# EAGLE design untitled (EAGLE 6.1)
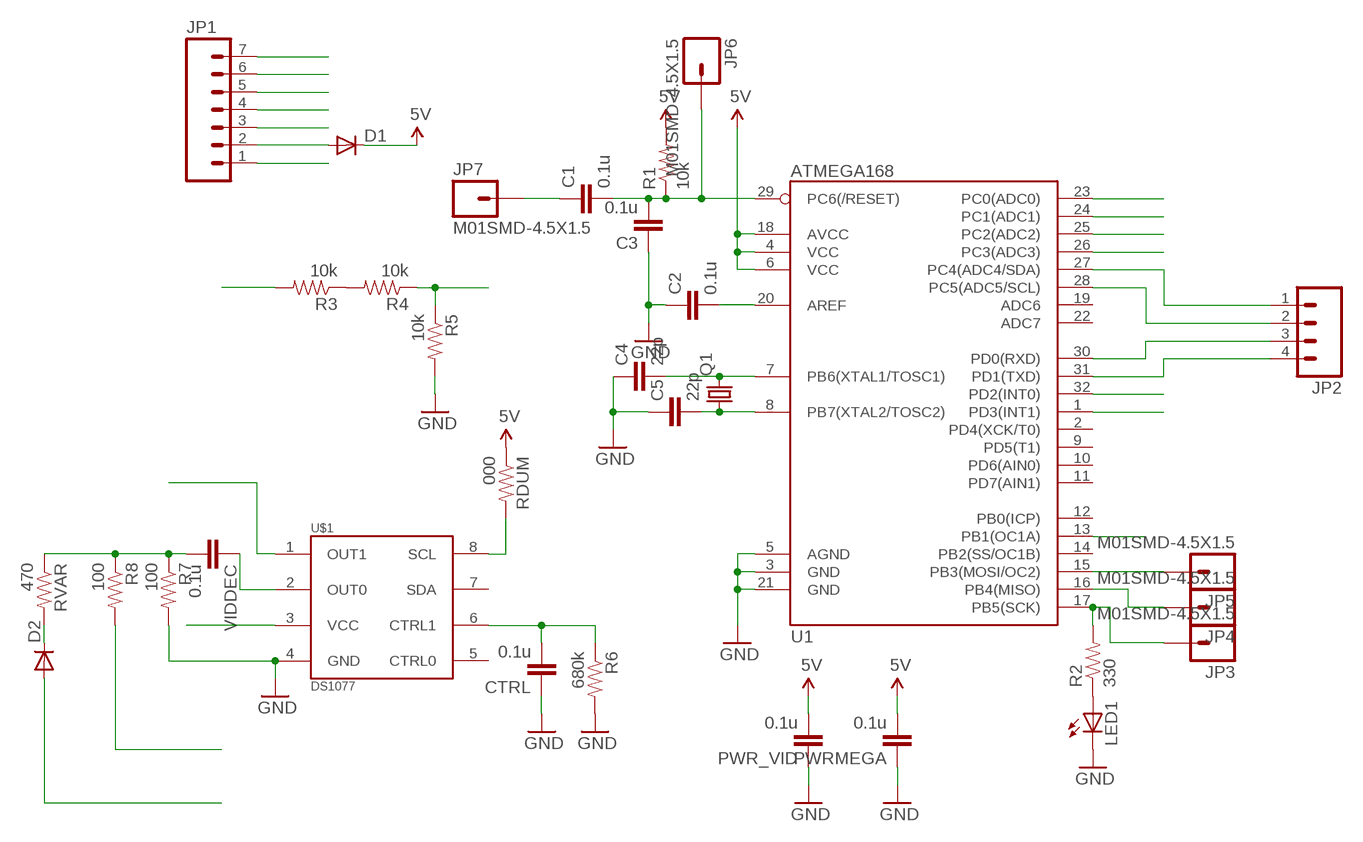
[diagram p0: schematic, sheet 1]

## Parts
C1  0.1u  CAP0805  [0805]
C2  0.1u  CAP0805  [0805]
C3  0.1u  CAP0805  [0805]
C4  22p  CAP0805  [0805]
C5  22p  CAP0805  [0805]
CTRL  0.1u  CAP0805  [0805]
D1  DIODESMA  [SMA-DIODE]
D2  DIODESMA  [SMA-DIODE]
JP1  M07  [1X07]
JP2  M04PTH  [1X04]
JP3  M01SMD-4.5X1.5  [PAD-1.5X4.5]
JP4  M01SMD-4.5X1.5  [PAD-1.5X4.5]
JP5  M01SMD-4.5X1.5  [PAD-1.5X4.5]
JP6  M01SMD-4.5X1.5  [PAD-1.5X4.5]
JP7  M01SMD-4.5X1.5  [PAD-1.5X4.5]
LED1  LED1206  [LED-1206]
PWR_VID  0.1u  CAP0805  [0805]
PWRMEGA  0.1u  CAP0805  [0805]
Q1  CRYSTAL10.5X4.8  [CRYSTAL-SMD-10.5X4.8-2PIN]
R1  10k  RESISTOR1206  [1206]
R2  330  RESISTOR1206  [1206]
R3  10k  RESISTOR1206  [1206]
R4  10k  RESISTOR1206  [1206]
R5  10k  RESISTOR1206  [1206]
R6  680k  RESISTOR1206  [1206]
R7  100  RESISTOR1206  [1206]
R8  100  RESISTOR1206  [1206]
RDUM  000  RESISTOR1206  [1206]
RVAR  470  RESISTOR1206  [1206]
U1  ATMEGA168  [TQFP32-08]
U$1  DS1077  [SO08]
VIDDEC  0.1u  CAP0805  [0805]

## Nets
5V: D1.C PWR_VID.2 PWRMEGA.2 R1.2 RDUM.1 U1.4(VCC) U1.6(VCC) U1.18(AVCC)
ADC0: JP1.4 U1.23(PC0(ADC0))
ADC2: JP1.5 U1.25(PC2(ADC2))
ADC3: JP1.6 U1.26(PC3(ADC3))
GND: C2.1 C3.1 C4.1 C5.1 CTRL.1 JP1.3 LED1.C PWR_VID.1 PWRMEGA.1 R5.2 R6.2 R7.2 U1.3(GND) U1.5(AGND) U1.21(GND) U$1.4(GND)
M1: U1.1(PD3(INT1)) U$1.3(VCC)
M13: R8.2 U1.13(PB1(OC1A))
M15: D2.A JP5.P$1 U1.15(PB3(MOSI/OC2))
M32: U1.32(PD2(INT0)) U$1.1(OUT1)
N$1: C2.2 U1.20(AREF)
N$2: C1.2 C3.2 JP6.P$1 R1.1 U1.29(PC6(/RESET))
N$3: C4.2 Q1.P$2 U1.7(PB6(XTAL1/TOSC1))
N$4: C5.2 Q1.P$1 U1.8(PB7(XTAL2/TOSC2))
N$5: JP2.1 U1.27(PC4(ADC4/SDA))
N$6: JP2.2 U1.28(PC5(ADC5/SCL))
N$7: JP2.3 U1.30(PD0(RXD))
N$8: JP2.4 U1.31(PD1(TXD))
N$9: LED1.A R2.1
N$10: JP3.P$1 R2.2 U1.17(PB5(SCK))
N$11: R3.1 R4.2
N$12: D1.A JP1.2
N$13: U$1.2(OUT0) VIDDEC.1
N$14: C1.1 JP7.P$1
N$15: RDUM.2 U$1.8(SCL)
N$16: JP4.P$1 U1.16(PB4(MISO))
N$19: CTRL.2 R6.1 U$1.6(CTRL1)
N$20: D2.C RVAR.2
VBAT: JP1.7 R3.2
VBAT_DIV: R4.1 R5.1 U1.24(PC1(ADC1))
VIDEOIN: JP1.1 R7.1 R8.1 RVAR.1 VIDDEC.2
Unconnected: U1.2(PD4(XCK/T0)) U1.9(PD5(T1)) U1.10(PD6(AIN0)) U1.11(PD7(AIN1)) U1.12(PB0(ICP)) U1.14(PB2(SS/OC1B)) U1.19(ADC6) U1.22(ADC7) U$1.5(CTRL0) U$1.7(SDA)

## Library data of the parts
C1-C5 CTRL PWR_VID PWRMEGA VIDDEC = SparkFun:CAP: Capacitor
D1 D2 = SparkFun:DIODE: Diode
JP1 = SparkFun:M07: Header 7 Standard 7-pin 0.1" header. Use with straight break away headers (SKU : PRT-00116), right angle break away headers (PRT-00553), swiss pins (PRT-00743), machine pins (PRT-00117), and female headers (PRT-00115). NOTES ON THE VARIANTS LOCK and LOCK_LONGPADS... This footprint was designed to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
JP2 = SparkFun:M04: Header 4 Standard 4-pin 0.1" header. Use with straight break away headers (SKU : PRT-00116), right angle break away headers (PRT-00553), swiss pins (PRT-00743), machine pins (PRT-00117), and female headers (PRT-00115). Molex polarized connector foot print use with SKU : PRT-08231 with associated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
JP3-JP7 = SparkFun:M01: Header 1
LED1 = SparkFun:LED: LEDs
Q1 = SparkFun:CRYSTAL: Crystals
R1-R8 RDUM RVAR = SparkFun:RESISTOR: Resistor
U1 = SparkFun:ATMEGA168
U$1 = SparkFun:DS1077

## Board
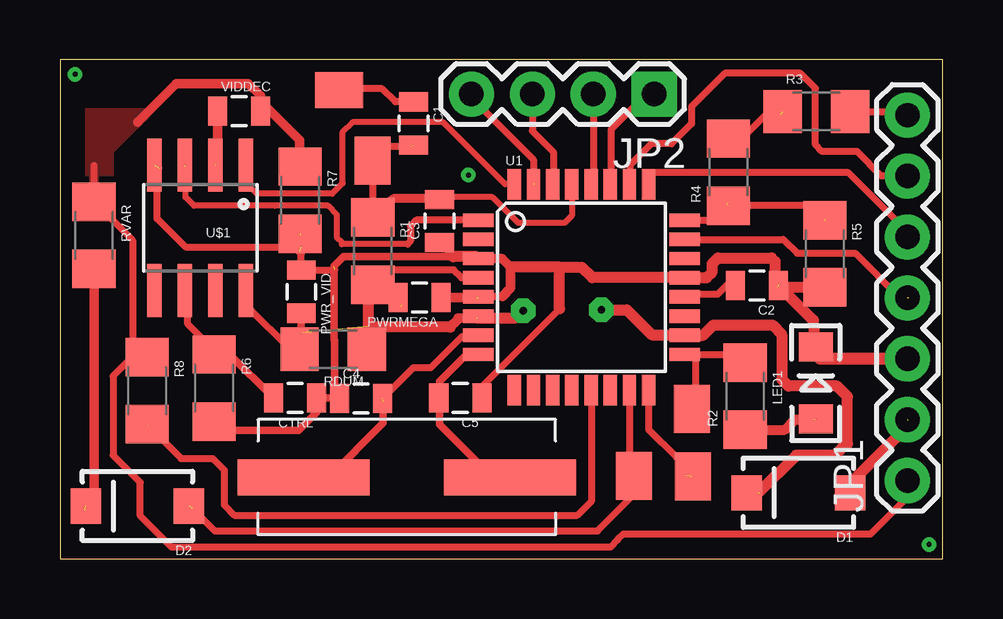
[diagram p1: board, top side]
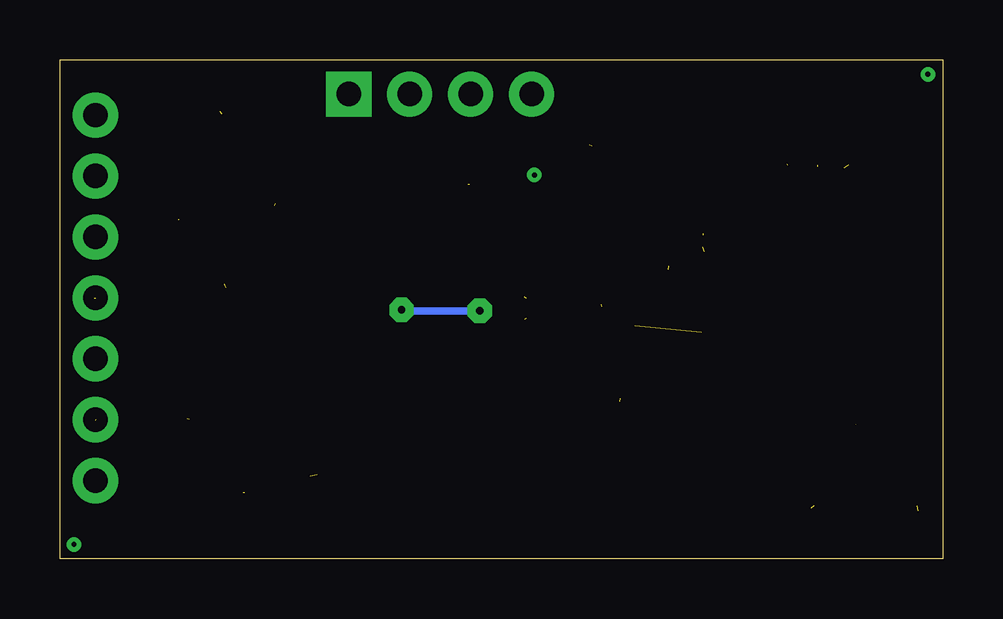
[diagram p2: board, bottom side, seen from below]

Size 36.81 x 20.8 mm. Coordinates in mm from the lower left corner, seen from the top.
Outline: 0,0 36.81,0 36.81,20.8 0,20.8 0,0
Copper layers (1*16): Top 0.035mm / dielectric 1.5mm / Bottom 0.035mm
Design rules: minimum track width 10mil, minimum drill 24mil, track to track 8mil, track to pad 8mil, pad to pad 8mil, via to via 8mil, smd to smd 8mil, copper to edge 40mil, drill to drill 8mil, minimum pad ring 10mil, minimum via ring 8mil, stop-mask expansion 4mil, vias tented up to drill 0mil, thermal gap 10mil

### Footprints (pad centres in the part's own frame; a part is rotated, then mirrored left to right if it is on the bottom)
0805 = smd 0.8 x 1.2: 1 -0.9,0; 2 0.9,0
SMA-DIODE = smd 1.27 x 1.47: A -2.15,0; C 2.15,0
1X07 = drill 1.016 pad 1.88: 1 0,0; 2 2.54,0; 3 5.08,0; 4 7.62,0; 5 10.16,0; 6 12.7,0; 7 15.24,0
1X04 = drill 1.016 pad 1.88 square: 1 0,0 | drill 1.016 pad 1.88: 2 2.54,0; 3 5.08,0; 4 7.62,0
PAD-1.5X4.5 = smd 1.5 x 2: P$1 0,0
LED-1206 = smd 1.2 x 1.4: A -1.5,0; C 1.5,0
CRYSTAL-SMD-10.5X4.8-2PIN = smd 5.5 x 1.5: P$1 -4.3,0; P$2 4.3,0
1206 = smd 1.6 x 1.8: 1 -1.4,0; 2 1.4,0
TQFP32-08 = smd 1.27 x 0.559: 1 -4.293,2.8; 2 -4.293,2; 3 -4.293,1.2; 4 -4.293,0.4; 5 -4.293,-0.4; 6 -4.293,-1.2; 7 -4.293,-2; 8 -4.293,-2.8; 17 4.293,-2.8; 18 4.293,-2; 19 4.293,-1.2; 20 4.293,-0.4; 21 4.293,0.4; 22 4.293,1.2; 23 4.293,2; 24 4.293,2.8 | smd 0.559 x 1.27: 9 -2.8,-4.293; 10 -2,-4.293; 11 -1.2,-4.293; 12 -0.4,-4.293; 13 0.4,-4.293; 14 1.2,-4.293; 15 2,-4.293; 16 2.8,-4.293; 25 2.8,4.293; 26 2,4.293; 27 1.2,4.293; 28 0.4,4.293; 29 -0.4,4.293; 30 -1.2,4.293; 31 -2,4.293; 32 -2.8,4.293
SO08 = smd 0.61 x 2.21: 1 -1.905,-2.616; 2 -0.635,-2.616; 3 0.635,-2.616; 4 1.905,-2.616; 5 1.905,2.616; 6 0.635,2.616; 7 -0.635,2.616; 8 -1.905,2.616

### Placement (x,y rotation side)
C1  14.74,18.15 270 top
C2  29.05,11.4 180 top
C3  15.82,14.08 90 top
C4  12.55,6.69 0 top
C5  16.69,6.71 180 top
CTRL  9.8,6.7 180 top
D1  30.78,2.75 180 top
D2  3.23,2.2 180 top
JP1  35.33,3.26 90 top
JP2  24.77,19.38 180 top
JP3  26.35,6.25 0 top
JP4  26.38,3.44 0 top
JP5  23.93,3.45 0 top
JP6  13.03,16.6 180 top
JP7  11.64,19.54 270 top
LED1  31.51,7.33 90 top
PWR_VID  10.06,11.14 270 top
PWRMEGA  14.99,10.9 180 top
Q1  14.46,3.4 180 top
R1  13.04,12.83 270 top
R2  28.56,6.78 90 top
R3  31.53,18.65 0 top
R4  27.86,16.12 90 top
R5  31.88,12.72 270 top
R6  6.43,7.12 270 top
R7  10.01,14.95 270 top
R8  3.63,7.01 270 top
RDUM  11.39,8.74 180 top
RVAR  1.42,13.49 270 top
U1  21.74,11.32 0 top
U$1  5.85,13.8 180 top
VIDDEC  7.47,18.66 0 top

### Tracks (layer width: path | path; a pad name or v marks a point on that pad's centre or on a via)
5V  (via drill 0.3 pad 1.02)  (4 unrouted)
  Top 0.3: D1.C 29.18,2.75 | 13.43,11.2 13.27,11.2 R1.2 13.04,11.83 13.27,12.06 13.75,12.06 13.77,12.04 16.41,12.04 16.73,11.72 U1.4 | 16.59,10.04 16.59,9.98 | 12.89,9.66 12.85,9.7
  Top 0.305: 17.43,10 17.63,10.2 | 17.37,10.04 U1.6 | 19.01,10.04 v19.31,10.34 | 26.01,9.34 U1.18 | 14.21,10.52 14.27,10.46 14.29,10.46 | 14.23,10.6 14.03,10.8 14.03,11 13.83,11.2 13.43,11.2 13.67,10.96 | PWRMEGA.2 13.67,10.96 | 13.67,10.96 13.13,10.96 12.85,10.68 | 12.85,9.7 12.85,9.48 RDUM.1 | PWR_VID.2 10.06,9.43 10.03,9.4
  Top 0.4: 16.59,10.04 17.37,10.04 | 16.59,9.98 16.27,9.66
  Top 0.45: U1.18 26.81,9.32 27.23,9.74 29.71,9.74 30.09,9.36 30.09,7.48 30.37,7.2 32.39,7.2 32.83,6.76 32.83,4.8 32.79,4.8 32.31,4.32 30.69,4.32 29.11,2.74 | 17.37,10.04 19.01,10.04 | v22.57,10.38 23.63,10.38 24.67,9.34 26.01,9.34 | 12.85,10.68 12.85,9.7 | 16.27,9.66 12.89,9.66
  Bottom 0.305: v19.31,10.34 22.53,10.34 v22.57,10.38
ADC0  (1 unrouted)
  Top 0.3: U1.23 30.15,13.32 30.73,12.74 33.15,12.74 35.01,10.88 35.39,10.88
ADC2
  Top 0.3: JP1.5 35.33,13.64 32.87,16.1 24.57,16.1 24.54,16.07 U1.25
ADC3
  Top 0.3: JP1.6 34.25,15.96 33.23,16.98 31.77,16.98 31.49,17.26 31.49,19.62 30.87,20.24 27.71,20.24 26.33,18.86 26.33,18.14 25.49,17.3 24.65,17.3 23.77,16.42 23.77,15.64 U1.26
GND  (7 unrouted)
  Top 0.22: 21.59,12.16 21.63,12.2 | 20.83,12.14 20.83,12.16
  Top 0.3: 29.67,12.54 29.81,12.4 | 29.81,11.62 29.97,11.46 | 11.45,12.06 11.43,12.04 PWR_VID.1 10.06,12.7 | 10.06,12.7 10.06,13.45 10.01,13.5 | 9.96,12.8 10.06,12.7 | 4.13,16.28 4.05,16.2 4.05,14.18 5.23,13 10.03,13 | 16.4,12.6 C3.1 | 31.68,8.34 LED1.C | 29.91,11.32 29.83,11.4 | 17.59,7.18 20.83,10.42 | 17.33,10.9 17.43,10.8
  Top 0.305: C5.1 17.59,7.18 | 17.53,11 U1.5 17.47,10.94 18.45,10.94 | 17.37,10.86 17.43,10.8 | 21.75,12.16 20.83,12.16 | U1.3 17.37,12.6 11.83,12.6 11.43,12.2 11.43,9.13 11.45,9.11 11.45,6.94 11.65,6.74 C4.1 11.62,6.69 11.61,6.7 CTRL.1 10.7,6.11 9.95,5.36 6.79,5.36 R6.2
  Top 0.4: U1.3 18.43,12.52 18.79,12.16 18.79,11.28 18.45,10.94 | PWRMEGA.1 17.33,10.9
  Top 0.45: 29.67,12.54 27.43,12.54 27.19,12.3 27.19,11.96 26.95,11.72 U1.21 22.19,11.72 21.75,12.16 | 29.81,12.4 29.81,11.62 | LED1.C 31.41,9.94 C2.1 | 18.79,12.16 20.83,12.16 21.59,12.16 | 17.37,12.6 16.4,12.6 | R5.2 29.91,11.32 | 20.83,10.42 20.83,12.14
  Top 0.5: JP1.3 31.68,8.34
M1  (1 unrouted)
  Top 0.22: 11.75,13.12 11.75,13.2
  Top 0.25: 11.75,13.2 11.55,13.4 11.55,14.34 11.17,14.72 8.95,14.72 5.59,14.72 5.23,15.08 5.23,16.34 5.21,16.36 | 14.49,13.12 11.75,13.12
  Top 0.3: U1.1 14.85,14.12 14.61,13.88 14.61,13.24 14.49,13.12
M13  (1 unrouted)
  Top 0.3: R8.2 | U1.13 22.17,7 22.17,2.42 21.57,1.82 7.27,1.82 6.85,2.24 6.85,3.7 6.37,4.18 5.05,4.18 R8.2
M15  (1 unrouted)
  Top 0.3: U1.15 23.74,3.64 JP5.P$1 23.97,3.41 23.97,2.72 22.41,1.16 6.45,1.16 5.5,2.11
M32
  Top 0.25: U$1.1 7.83,16.34 7.83,15.6 8.21,15.22 11.35,15.22 11.79,15.66 11.77,15.68 11.77,17.78 12.19,18.2 15.97,18.2 18.56,15.61 U1.32
N$1
  Top 0.3: C2.2 27.79,11.4 27.41,11.02 26.13,11.02 U1.20
N$2  (1 unrouted)
  Top 0.25: U1.29 21.34,14.31 21.03,14 19.11,14 18.03,15.08 13.89,15.08 13.44,14.63 R1.1
  Top 0.3: C3.2 13.79,14.98 13.44,14.63 | 14.63,17.2 13.23,17.2 13.03,17 JP6.P$1 R1.1
N$3  (1 unrouted)
  Top 0.3: 17.39,9.26 16.75,9.26 15.45,7.96 14.72,7.96 C4.2
  Top 0.305: Q1.P$2 11.21,3.4 13.47,5.66 13.47,6.56 | C4.2 13.54,6.69 | 17.39,9.26 U1.7
N$4
  Top 0.305: U1.8 16.95,8.52 15.83,7.4 15.83,6.75 C5.2 15.83,6.67 15.83,5.6 18.03,3.4 Q1.P$1
N$5
  Top 0.3: JP2.1 24.45,19.38 22.97,17.9 22.97,15.64 U1.27
N$6
  Top 0.3: JP2.2 22.23,15.7 U1.28
N$7
  Top 0.3: JP2.3 19.69,17.84 20.57,16.96 20.57,15.64 U1.30
N$8  (1 unrouted)
  Top 0.3: JP2.4 17.15,19.22 19.73,16.64 19.73,15.68 19.79,15.62
N$9  (1 unrouted)
  Top 0.406: R2.1 30.21,5.38 30.63,5.8 31.43,5.8
N$10
  Top 0.3: JP3.P$1 26.49,5.81 26.49,8.44 26.41,8.52 U1.17 28.52,8.52 R2.2
N$11  (1 unrouted)
  Top 0.3: R4.2 28.43,17.52 29.45,18.54 30.05,18.54
N$12  (1 unrouted)
  Top 0.3: 35.19,5.6 35.35,5.76
  Top 0.45: D1.A 32.93,3.12 34.95,5.14 34.95,5.42 JP1.2
N$13  (1 unrouted)
  Top 0.3: 6.57,16.52 6.51,16.46
  Top 0.4: VIDDEC.1 6.57,16.52
N$14
  Top 0.3: C1.1 13.98,19.05 13.43,19.6 11.7,19.6 JP7.P$1
N$15
  Top 0.3: RDUM.2 9.59,8.74 7.87,10.46 7.87,11.05 U$1.8
N$16  (1 unrouted)
  Top 0.3: U1.16 24.54,5.39 25.69,4.24 26.07,3.84 26.09,3.5
N$17
  Top 0.305: 6.83,8.4 6.23,8.4 6.23,8.6
N$18  (via drill 0.2)
  other vias: 0.63,20.2
N$19
  Top 0.3: R6.1 6.43,8.68 5.33,9.78 5.33,11.05 U$1.6
  Top 0.305: R6.1 7.08,8.52 CTRL.2
N$20  (1 unrouted)
  Top 0.3: 1.42,2.19 1.23,2 1.03,2
  Top 0.4: RVAR.2 1.42,2.19
N$21  (via drill 0.2)
  other vias: 17.03,16
N$181  (via drill 0.2)
  other vias: 36.23,0.6
VBAT
  Top 0.3: R3.2 35.18,18.65 JP1.7
VBAT_DIV  (2 unrouted)
  Top 0.3: U1.24 28.15,14.12 | 28.15,14.12 28.77,14.74 31.27,14.74 31.87,14.14 | 28.15,14.12 28.15,14.48 27.83,14.8
VIDEOIN
  Top 0.3: 1.41,16.4 RVAR.1 3.03,13.28 3.03,9.01 R8.1 3,8.41 2.21,7.62 2.21,4.32 3.35,3.18 3.35,1.78 4.65,0.48 22.95,0.48 23.25,0.78 23.25,0.8 23.47,1.02 33.79,1.02 35.33,2.56 JP1.1 | VIDDEC.2 8.59,18.86 | 9.99,16.37 R7.1
  Top 0.4: 8.59,18.86 9.99,17.46 9.99,16.37 | VIDDEC.2 8.37,19.3 7.85,19.82 4.85,19.82 3.23,18.2
  pour Top: 0.83,15 0.83,18.6 3.63,18.6 2.03,17 2.03,15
